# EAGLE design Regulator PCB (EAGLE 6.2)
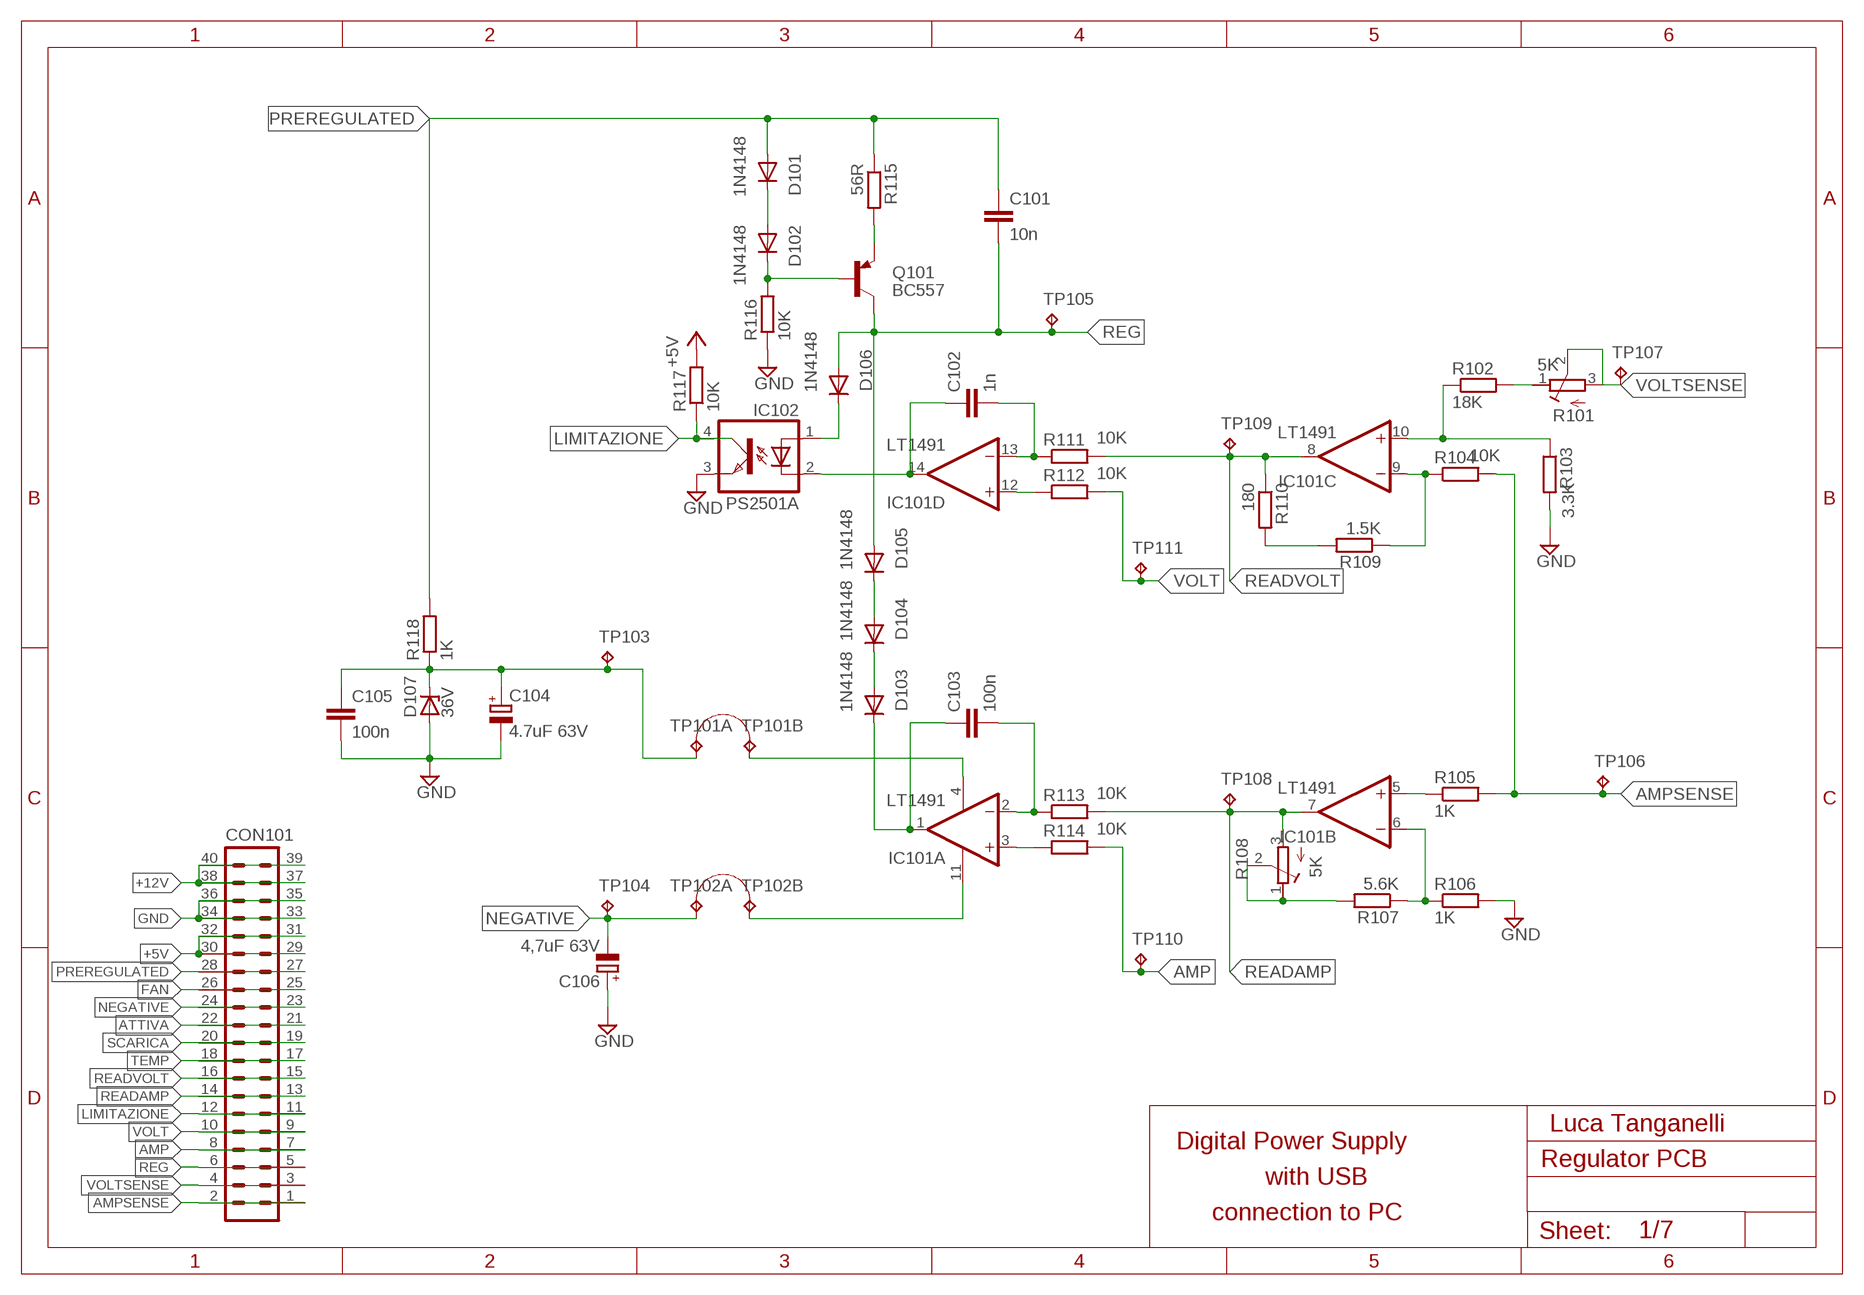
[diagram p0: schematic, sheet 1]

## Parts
C101  10n  C-EU050-024X044  [C050-024X044]
C102  1n  C-EU050-024X044  [C050-024X044]
C103  100n  C-EU050-024X044  [C050-024X044]
C104  4.7uF 63V  CPOL-EUE2.5-5  [E2,5-5]
C105  100n  C-EU050-024X044  [C050-024X044]
C106  4,7uF 63V  CPOL-EUE2.5-5  [E2,5-5]
CON101  ML40  [ML40]
D101  1N4148  1N4148DO35-7  [DO35-7]
D102  1N4148  1N4148DO35-7  [DO35-7]
D103  1N4148  1N4148DO35-10  [DO35-10]
D104  1N4148  1N4148DO35-10  [DO35-10]
D105  1N4148  1N4148DO35-10  [DO35-10]
D106  1N4148  1N4148DO35-10  [DO35-10]
D107  36V  1N4728  [DO41Z10]
IC101  LT1491  TL084P  [DIL14]
IC102  PS2501A  TIL191  [DIL04]
Q101  BC557  [TO92-EBC]
R101  5K  R-TRIMMT93YA  [RTRIMT93YA]
R102  18K  R-EU_0207/10  [0207/10]
R103  3.3K  R-EU_0207/10  [0207/10]
R104  10K  R-EU_0207/12  [0207/12]
R105  1K  R-EU_0207/10  [0207/10]
R106  1K  R-EU_0207/10  [0207/10]
R107  5.6K  R-EU_0207/10  [0207/10]
R108  5K  R-TRIMMT93YA  [RTRIMT93YA]
R109  1.5K  R-EU_0207/10  [0207/10]
R110  180  R-EU_0207/10  [0207/10]
R111  10K  R-EU_0207/12  [0207/12]
R112  10K  R-EU_0207/10  [0207/10]
R113  10K  R-EU_0207/10  [0207/10]
R114  10K  R-EU_0207/10  [0207/10]
R115  56R  R-EU_0207/10  [0207/10]
R116  10K  R-EU_0207/10  [0207/10]
R117  10K  R-EU_0207/10  [0207/10]
R118  1K  R-EU_0309/12  [0309/12]
TP101  TP2  [TP2]
TP102  TP2  [TP2]
TP103  TP  [TP1]
TP104  TP  [TP1]
TP105  TP  [TP1]
TP106  TP  [TP1]
TP107  TP  [TP1]
TP108  TP  [TP1]
TP109  TP  [TP1]
TP110  TP  [TP1]
TP111  TP  [TP1]

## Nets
+5V: CON101.29 CON101.30 CON101.31 CON101.32 R117.2
+12V: CON101.37 CON101.38 CON101.39 CON101.40
AMP: CON101.7 CON101.8 R114.2 TP110.P$1(TP)
AMPSENSE: CON101.1 CON101.2 R104.2 R105.2 TP106.P$1(TP)
ATTIVA: CON101.21 CON101.22
FAN: CON101.25 CON101.26
GND: C104.- C105.2 C106.+ CON101.33 CON101.34 CON101.35 CON101.36 D107.A IC102.3(EMIT) R103.2 R106.2 R116.1
LIMITAZIONE: CON101.11 CON101.12 IC102.4(COL) R117.1
N$1: IC101.5(B:+IN) R105.1
N$2: IC101.6(B:-IN) R106.1 R107.1
N$3: IC101.10(C:+IN) R102.1 R103.1
N$4: IC101.9(C:-IN) R104.1 R109.1
N$5: C102.2 IC101.13(D:-IN) R111.1
N$6: IC101.12(D:+IN) R112.1
N$7: C103.2 IC101.2(A:-IN) R113.1
N$8: IC101.3(A:+IN) R114.1
N$9: R107.2 R108.1(A) R108.2(S)
N$10: IC101.4(P:V+) TP101.P$2
N$11: D103.A D104.C
N$13: R101.1(A) R102.2
N$14: R109.2 R110.2
N$17: C102.1 IC101.14(D:OUT) IC102.2(C)
N$18: C103.1 D103.C IC101.1(A:OUT)
N$20: Q101.E R115.2
N$21: D101.C D102.A
N$22: D102.C Q101.B R116.2
N$23: C104.+ C105.1 D107.C R118.1 TP101.P$1 TP103.P$1(TP)
N$24: D104.A D105.C
N$26: D106.C IC102.1(A)
N$29: IC101.11(P:V-) TP102.P$2
NEGATIVE: C106.- CON101.23 CON101.24 TP102.P$1 TP104.P$1(TP)
PREREGULATED: C101.1 CON101.27 CON101.28 D101.A R115.1 R118.2
READAMP: CON101.13 CON101.14 IC101.7(B:OUT) R108.3(E) R113.2 TP108.P$1(TP)
READVOLT: CON101.15 CON101.16 IC101.8(C:OUT) R110.1 R111.2 TP109.P$1(TP)
REG: C101.2 CON101.5 CON101.6 D105.A D106.A Q101.C TP105.P$1(TP)
SCARICA: CON101.19 CON101.20
TEMP: CON101.17 CON101.18
VOLT: CON101.9 CON101.10 R112.2 TP111.P$1(TP)
VOLTSENSE: CON101.3 CON101.4 R101.2(S) R101.3(E) TP107.P$1(TP)

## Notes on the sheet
- Luca Tanganelli
- Digital Power Supply
- with USB
- connection to PC
- 1/7

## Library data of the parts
C101-C103 C105 = #-rcl:C-EU: CAPACITOR, European symbol
C104 C106 = #-rcl:CPOL-EU: POLARIZED CAPACITOR, European symbol
CON101 = #-con-ml:ML40: HARTING; OC_FARNELL: unknown; OC_NEWARK: unknown
D101-D106 = #-diode:1N4148: DIODE
D107 = #-diode:1N4728: Z DIODE
IC101 = #-linear:TL084: OP AMP
IC102 = #-optocoupler:TIL191: TEXAS INSTRUMENTS OPTO COUPLER; OC_FARNELL: 1683363; OC_NEWARK: unknown
Q101 = #-transistor-pnp:BC557*: PNP Transistror
R101 R108 = #-rcl:R-TRIMM: Trimm resistor
R102-R107 R109-R118 = #-rcl:R-EU_: RESISTOR, European symbol
TP101 TP102 = #-testpad:TP2: Test pad
TP103-TP111 = #-testpad:TP: Test pad

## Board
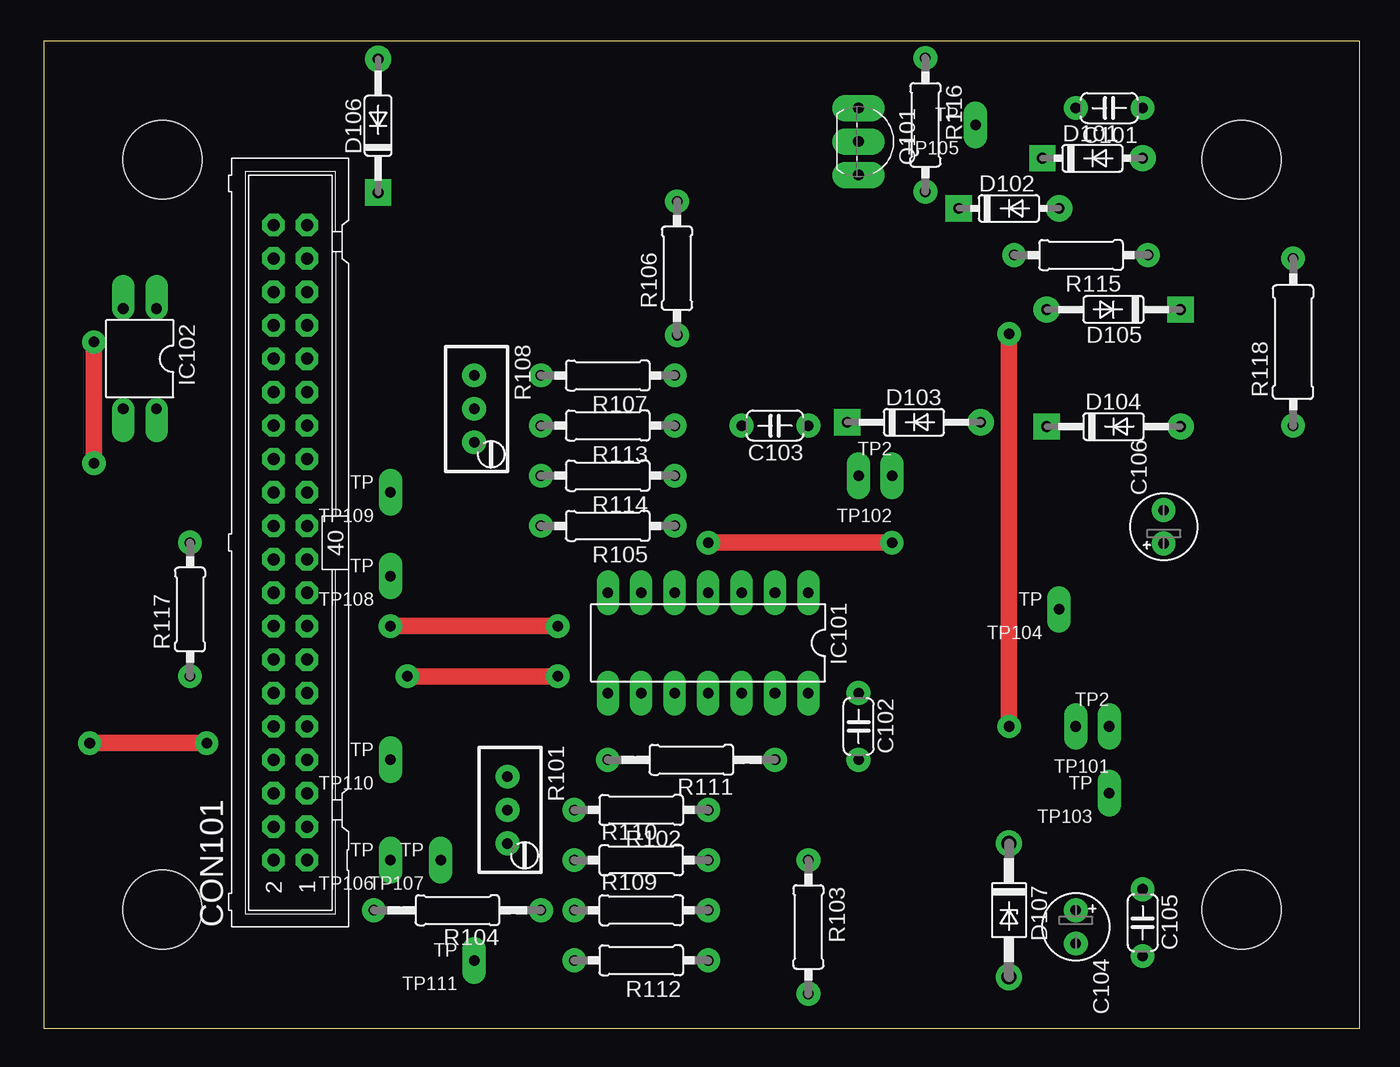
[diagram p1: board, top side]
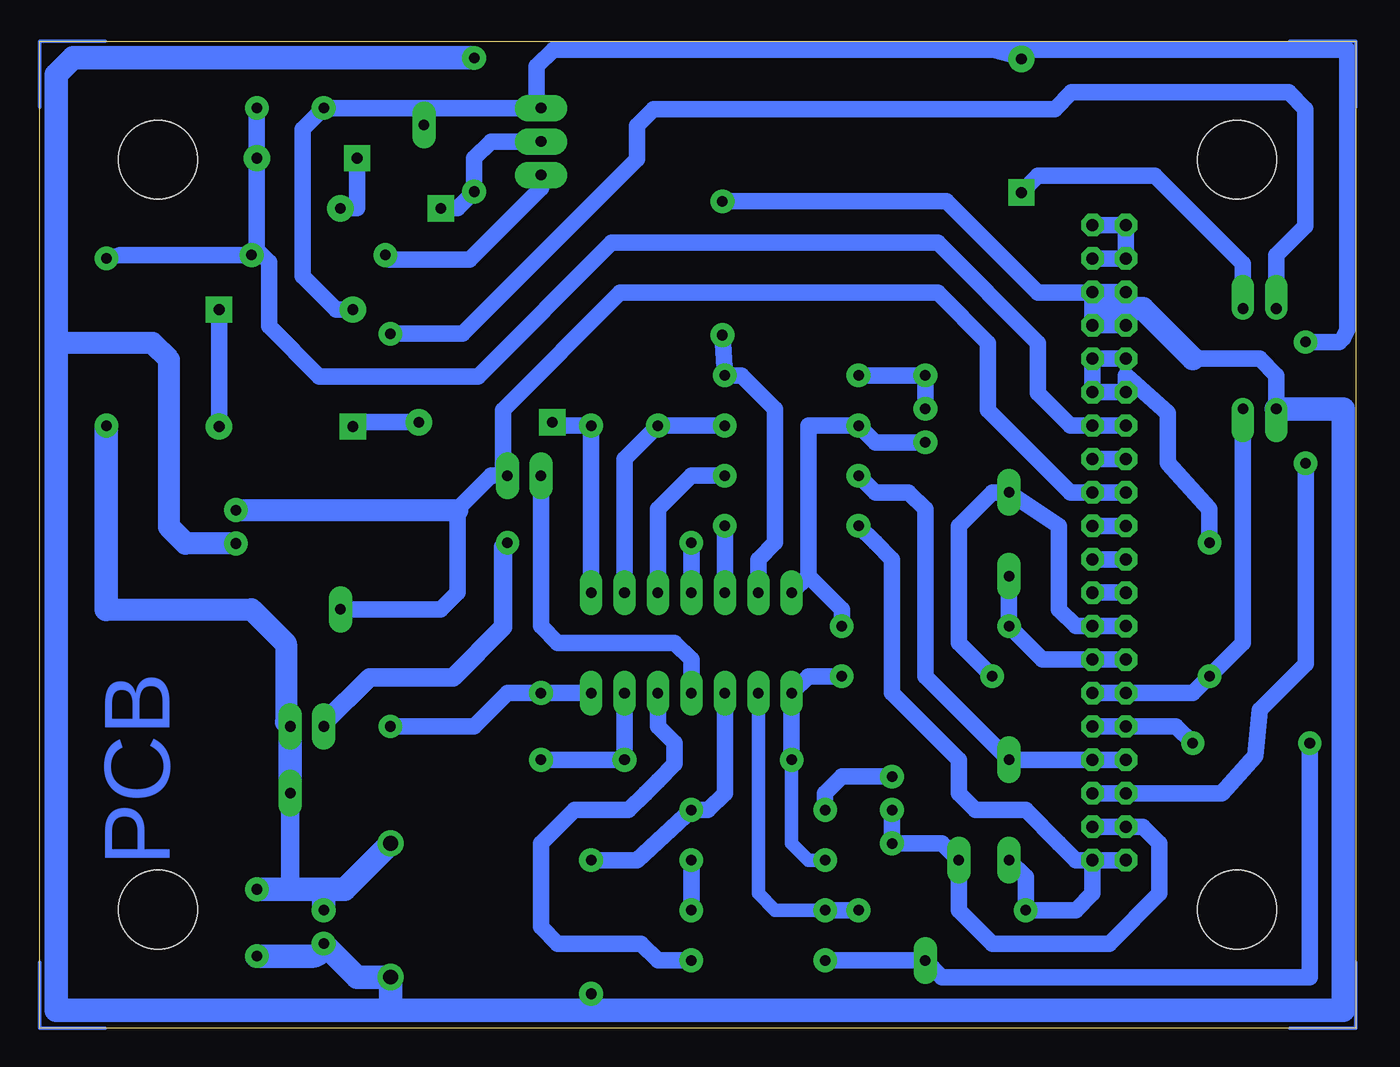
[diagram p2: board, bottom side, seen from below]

Size 100 x 75 mm. Coordinates in mm from the lower left corner, seen from the top.
Outline: 100,75 0,75 0,0 100,0 100,75
Copper layers (1*16): Top 0.035mm / dielectric 1.5mm / Bottom 0.035mm
Design rules: minimum track width 10mil, minimum drill 24mil, track to track 8mil, track to pad 8mil, pad to pad 8mil, via to via 8mil, smd to smd 8mil, copper to edge 40mil, drill to drill 8mil, minimum pad ring 10mil, minimum via ring 8mil, stop-mask expansion 4mil, vias tented up to drill 0mil, thermal gap 10mil
Holes 6 mm at 91,9 91,66 9,66 9,9

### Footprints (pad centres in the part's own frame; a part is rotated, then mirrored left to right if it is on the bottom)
C050-024X044 = drill 0.8 pad 1.8: 1 -2.54,0; 2 2.54,0
E2,5-5 = drill 0.8 pad 1.8: + -1.27,0; - 1.27,0
ML40 = drill 0.914 pad 1.7 octagon: 1 -24.13,-1.27; 2 -24.13,1.27; 3 -21.59,-1.27; 4 -21.59,1.27; 5 -19.05,-1.27; 6 -19.05,1.27; 7 -16.51,-1.27; 8 -16.51,1.27; 9 -13.97,-1.27; 10 -13.97,1.27; 11 -11.43,-1.27; 12 -11.43,1.27; 13 -8.89,-1.27; 14 -8.89,1.27; 15 -6.35,-1.27; 16 -6.35,1.27; 17 -3.81,-1.27; 18 -3.81,1.27; 19 -1.27,-1.27; 20 -1.27,1.27; 21 1.27,-1.27; 22 1.27,1.27; 23 3.81,-1.27; 24 3.81,1.27; 25 6.35,-1.27; 26 6.35,1.27; 27 8.89,-1.27; 28 8.89,1.27; 29 11.43,-1.27; 30 11.43,1.27; 31 13.97,-1.27; 32 13.97,1.27; 33 16.51,-1.27; 34 16.51,1.27; 35 19.05,-1.27; 36 19.05,1.27; 37 21.59,-1.27; 38 21.59,1.27; 39 24.13,-1.27; 40 24.13,1.27
DO35-7 = drill 0.813 pad 2: A 3.81,0 | drill 0.813 pad 2 square: C -3.81,0
DO35-10 = drill 0.813 pad 2: A 5.08,0 | drill 0.813 pad 2 square: C -5.08,0
DO41Z10 = drill 1.118 pad 2: A 5.08,0; C -5.08,0
DIL14 = drill 0.8 pad 1.7 long: 1 -7.62,-3.81; 2 -5.08,-3.81; 3 -2.54,-3.81; 4 0,-3.81; 5 2.54,-3.81; 6 5.08,-3.81; 7 7.62,-3.81; 8 7.62,3.81; 9 5.08,3.81; 10 2.54,3.81; 11 0,3.81; 12 -2.54,3.81; 13 -5.08,3.81; 14 -7.62,3.81
DIL04 = drill 0.813 pad 1.7 offset: 1 -1.27,-3.81; 2 1.27,-3.81; 3 1.27,3.81; 4 -1.27,3.81
TO92-EBC = drill 0.813 pad 2 long: B 0,-1.27; C -2.54,-1.27; E 2.54,-1.27
RTRIMT93YA = drill 0.8 pad 1.8: 1 0,-2.54; 2 0,0; 3 0,2.54
0207/10 = drill 0.8 pad 1.8: 1 -5.08,0; 2 5.08,0
0207/12 = drill 0.8 pad 1.8: 1 -6.35,0; 2 6.35,0
0309/12 = drill 0.8 pad 1.8: 1 -6.35,0; 2 6.35,0
TP2 = drill 0.8 pad 1.778 long: P$1 -1.27,0; P$2 1.27,0
TP1 = drill 0.8 pad 1.778 long: P$1 0,0

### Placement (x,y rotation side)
C101  80.95,69.92 180 top
C102  61.9,22.93 270 top
C103  55.55,45.79 180 top
C104  78.41,7.69 270 top
C105  83.49,8.01 270 top
C106  85.09,38.1 90 top
CON101  18.72,36.9 90 top
D101  79.68,66.11 0 top
D102  73.33,62.3 0 top
D103  66.11,46.05 0 top
D104  81.28,45.72 0 top
D105  81.28,54.61 180 top
D106  25.4,68.58 90 top
D107  73.33,8.96 270 top
IC101  50.47,29.28 180 top
IC102  7.29,50.87 180 top
Q101  63.17,67.38 270 top
R101  35.23,16.58 180 top
R102  45.39,16.58 180 top
R103  58.09,7.69 270 top
R104  31.42,8.96 180 top
R105  42.85,38.17 180 top
R106  48.11,57.75 90 top
R107  42.85,49.6 180 top
R108  32.69,47.06 180 top
R109  45.39,8.96 0 top
R110  45.39,12.77 0 top
R111  49.2,20.39 180 top
R112  45.39,5.15 180 top
R113  42.85,45.79 180 top
R114  42.85,41.98 180 top
R115  78.81,58.75 180 top
R116  66.98,68.65 270 top
R117  11.1,31.82 90 top
R118  94.92,52.14 90 top
TP101  79.68,22.93 180 top
TP102  63.17,41.98 180 top
TP103  80.95,17.85 180 top
TP104  77.14,31.82 180 top
TP105  70.79,68.65 180 top
TP106  26.34,12.77 180 top
TP107  30.15,12.77 180 top
TP108  26.34,34.36 180 top
TP109  26.34,40.71 180 top
TP110  26.34,20.39 180 top
TP111  32.69,5.15 180 top

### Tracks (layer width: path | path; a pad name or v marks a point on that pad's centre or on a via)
+5V
  Bottom 1.27: R117.2 11.1,39.44 14.28,42.93 14.28,46.74 17.45,49.6 CON101.30 CON101.29 CON101.31 CON101.32
+12V
  Bottom 1.27: CON101.39 CON101.40 CON101.38 CON101.37
AMP
  Bottom 1.27: CON101.8 CON101.7 TP110.P$1 32.69,26.74 32.69,39.44 33.96,40.71 36.5,40.71 R114.2
AMPSENSE
  Bottom 1.27: CON101.2 CON101.1 | R105.2 36.5,36.9 35.23,35.63 35.23,25.47 30.15,20.39 30.15,17.85 28.88,16.58 25.07,16.58 22.53,14.04 21.26,12.77 CON101.1 | CON101.1 19.99,10.23 21.26,8.96 R104.2 25.07,11.5 TP106.P$1
ATTIVA
  Bottom 1.27: CON101.21 CON101.22
FAN
  Bottom 1.27: CON101.25 CON101.26
GND
  Bottom 1.27: CON101.33 CON101.34 18.72,54.68 19.99,54.68 CON101.33 | CON101.36 CON101.35 | CON101.33 CON101.35 | IC102.3 6.02,49.6 7.29,50.87 12.37,50.87 | R103.2 58.09,1.34 | R106.2 31.08,62.83 24.13,55.88 20.06,55.88 CON101.35
  Bottom 1.676: C106.+ 88.9,36.83 90.17,38.1 90.17,50.8 91.44,52.07 98.73,52.07
  Bottom 1.778: R116.1 97.46,73.73 98.73,72.46 98.73,52.07 98.73,1.34 73.33,1.34 | 12.37,50.87 16.18,54.68 18.72,54.68 | C105.2 79.36,5.47 arc-90 C104.- 75.87,3.88 D107.A 73.33,1.34 | 73.33,1.34 58.09,1.34 0.94,1.34 0.94,47.06 IC102.3
LIMITAZIONE
  Bottom 1.27: CON101.11 CON101.12 12.37,25.47 R117.1 8.56,29.28 8.56,40.71 8.56,43.25 IC102.4
N$1
  Bottom 1.27: R105.1 47.93,36.9 IC101.5
N$2
  Bottom 1.27: R106.1 R107.1 46.66,49.6 44.12,47.06 44.12,36.9 45.39,35.63 IC101.6
N$3
  Bottom 1.27: IC101.10 47.93,17.85 49.2,16.58 R102.1 54.6,12.77 R103.1
N$4
  Bottom 1.016: IC101.9 45.39,10.23 44.12,8.96 R109.1
  Bottom 1.27: R109.1 R104.1
N$5
  Bottom 1.27: IC101.13 55.55,21.66 R111.1 C102.2
N$6
  Bottom 1.27: IC101.12 53.01,22.93 51.74,21.66 51.74,20.07 53.01,18.8 53.96,17.85 55.23,16.58 59.36,16.58 61.9,14.04 61.9,7.69 60.63,6.42 54.28,6.42 53.01,5.15 R112.1
N$7
  Bottom 1.27: IC101.2 55.55,43.25 C103.2 R113.1
N$8
  Bottom 1.27: R114.1 50.47,41.98 53.01,39.44 53.01,35.63 IC101.3
N$9
  Bottom 1.27: R107.2 R108.1 R108.2
N$10  (via drill 0.8 pad 1.78)
  Top 1.27: v50.47,36.9 v64.44,36.9
  Bottom 1.27: IC101.4 v50.47,36.9
  Bottom 1.422: TP101.P$2 78.41,23.19 74.93,26.67 68.58,26.67 64.77,30.48 64.77,36.57 v64.44,36.9
N$11
  Bottom 1.27: D104.C 75.87,46.05 D103.A
N$12
  Bottom 0.254: 100,70 100,75 95,75
N$13
  Bottom 1.27: R102.2 40.31,17.85 39.04,19.12 37.77,19.12 36.5,19.12 R101.1
N$14
  Bottom 1.27: R110.2 R109.2
N$15
  Bottom 0.254: 5,75 0,75 0,70
N$16
  Bottom 0.254: 5,0 0,0 0,5
N$17  (via drill 0.8 pad 1.78)
  Top 1.27: v73.33,52.77 v73.33,22.93
  Bottom 1.27: 6.02,58.49 IC102.2 6.02,58.75 3.81,60.96 3.81,69.85 5.08,71.12 21.59,71.12 22.86,69.85 53.34,69.85 54.61,68.58 54.61,66.04 67.88,52.77 v73.33,52.77 | IC101.14 C102.1 64.44,25.47 66.98,22.93 v73.33,22.93
N$18
  Bottom 1.27: IC101.1 C103.1 60.77,45.79 D103.C
N$19
  Bottom 0.254: 100,5 100,0 95,0
N$20
  Bottom 1.27: Q101.E 61.9,63.83 67.31,58.42 73.4,58.42 R115.2
N$21
  Bottom 1.27: D101.C 75.87,62.3 D102.A
N$22
  Bottom 1.27: Q101.B 65.71,67.38 66.98,66.11 R116.2 68.25,62.3 D102.C
N$23
  Bottom 1.422: TP103.P$1 80.95,10.88 81.28,10.55
  Bottom 1.676: 94.92,31.82 83.89,31.82 81.28,29.21 81.28,23.26 TP101.P$1
  Bottom 1.778: R118.1 94.92,31.82 | D107.C 76.82,10.55 78.41,10.55 | 78.41,10.55 81.28,10.55 C105.1 | C104.+ 78.41,10.55 | TP101.P$1 TP103.P$1
N$24
  Bottom 1.27: D105.C D104.A
N$25  (via drill 1 pad 2.54)
  other vias: 91,9
N$26
  Bottom 1.27: D106.C 24.13,64.77 15.24,64.77 8.56,58.09 IC102.1
N$29
  Bottom 1.27: IC101.11 50.47,28.01 51.74,29.28 60.63,29.28 61.9,30.55 61.9,40.71 TP102.P$2
N$31  (via drill 1 pad 2.54)
  other vias: 9,9
N$32  (via drill 1 pad 2.54)
  other vias: 9,66
N$33  (via drill 1 pad 2.54)
  other vias: 91,66
NEGATIVE
  Bottom 1.27: CON101.24 CON101.23 21.66,40.71 27.94,46.99 27.94,52.07 31.75,55.88 55.88,55.88 64.77,46.99 64.77,42.31 TP102.P$1 65.71,41.98 68.25,39.44 68.25,39.37 68.25,33.09 69.52,31.82 TP104.P$1
  Bottom 1.676: C106.- 68.25,39.37
PREREGULATED
  Bottom 1.27: CON101.28 CON101.27 21.66,45.79 24.13,48.26 24.13,52.07 31.75,59.69 56.52,59.69 66.68,49.53 78.74,49.53 82.55,53.34 82.55,58.21 83.49,59.15 | C101.1 D101.A 83.49,59.15 | 83.49,59.15 R115.1 93.91,58.75 R118.2
READAMP  (via drill 0.8 pad 1.78)
  Top 1.27: v39.04,30.55 v26.34,30.55
  Bottom 1.27: CON101.14 CON101.13 23.8,28.01 v26.34,30.55 TP108.P$1 | 41.58,34.36 41.58,45.79 R113.2 36.5,44.52 R108.3 | 41.58,34.36 IC101.7 | 41.58,34.36 39.04,31.82 v39.04,30.55
READVOLT  (via drill 0.8 pad 1.78)
  Top 1.27: v39.04,26.74 v27.61,26.74
  Bottom 1.016: R111.2 42.85,14.04 41.58,12.77 R110.1
  Bottom 1.27: CON101.16 CON101.15 21.26,30.55 22.53,31.82 22.53,38.17 TP109.P$1 27.61,40.71 30.15,38.17 30.15,29.28 v27.61,26.74 | R111.2 IC101.8 41.58,26.74 v39.04,26.74
REG  (via drill 0.8 pad 1.78)
  Top 1.27: v3.8,42.93 v3.8,52.14
  Bottom 1.016: D106.A 27.94,74.36
  Bottom 1.27: 70.79,69.92 C101.2 80.01,68.32 80.01,57.15 77.47,54.61 D105.A | 70.79,69.92 Q101.C 62.18,70 62.18,69.9 62.23,69.85 62.23,73.09 60.96,74.36 27.94,74.36 0.62,74.36 0.62,53.09 0.94,52.46 1.26,52.14 v3.8,52.14 | CON101.6 CON101.5 10.15,17.85 7.61,20.71 7.29,24.2 3.8,27.69 v3.8,42.93 | TP105.P$1 70.79,69.92
SCARICA
  Bottom 1.27: CON101.19 CON101.20
TEMP
  Bottom 1.27: CON101.17 CON101.18
VOLT  (via drill 0.8 pad 1.78)
  Top 1.27: v3.48,21.66 v12.37,21.66
  Bottom 1.27: CON101.9 CON101.10 13.64,22.93 v12.37,21.66 | R112.2 TP111.P$1 31.42,3.88 17.45,3.88 3.48,3.88 v3.48,21.66
VOLTSENSE
  Bottom 1.27: CON101.3 18.72,15.31 CON101.4 16.18,15.31 14.91,14.04 14.91,10.23 18.72,6.42 27.61,6.42 30.15,8.96 TP107.P$1 31.42,14.04 R101.3 R101.2

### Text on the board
Bottom: PCB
